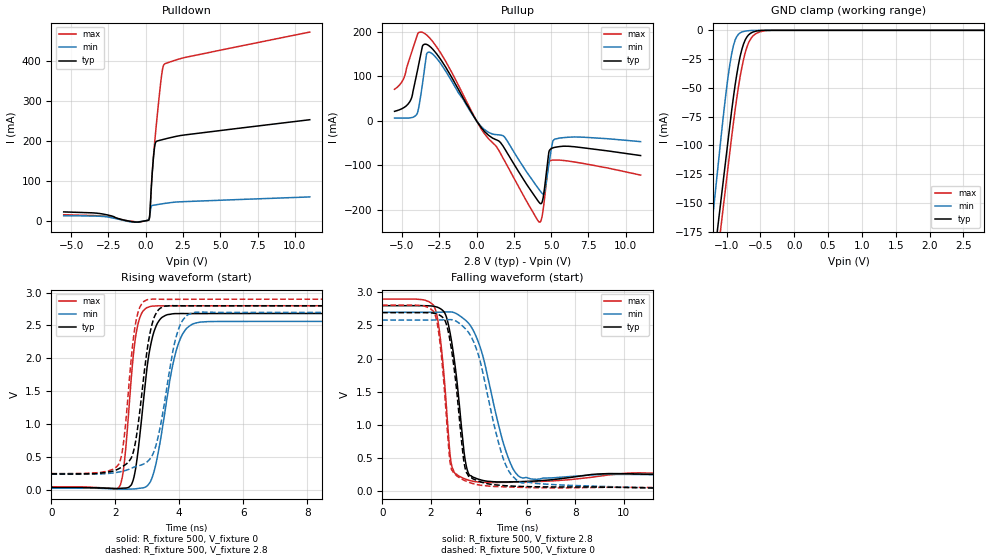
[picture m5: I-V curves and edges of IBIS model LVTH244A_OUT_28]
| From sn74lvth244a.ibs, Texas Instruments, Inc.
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[Model]   LVTH244A_OUT_28
Model_type  3-state
Enable   Active-Low
Vref =   0
Rref =   500
Cref =   50p
Vmeas =   1.5
| variable   typ   min   max
C_comp   5.78pF   4.77pF   7.95pF
| C_pullup   4.85pF   0.29pF   7.49pF
| C_pulldown   5.95pF   2.16pF   9.97pF
| C_tri-state   5.78pF   4.77pF   7.95pF
[Temperature Range]   40   -40   100
| Ambient temperature   25   -40   85
[Voltage range]   2.8   2.7   2.9
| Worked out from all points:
|   slope of the pulldown table from 0 to 0.42 V, typ, clamps not added: 3.84 ohm
|   slope of the pullup table from 0 to 0.42 V, typ, clamps not added: 21.7 ohm
|   GND clamp passes 1 mA (typ) near -0.58 V on its own axis
|   rising waveform, R_fixture 500, V_fixture 0: 20-80 % time 381ps typ, 543ps min, 293ps max; typ from 0.032 V to 2.68 V
|   falling waveform, R_fixture 500, V_fixture 2.8: 20-80 % time 483ps typ, 987ps min, 372ps max; typ from 2.8 V to 0.238 V
|   rising waveform, R_fixture 500, V_fixture 2.8: 20-80 % time 408ps typ, 541ps min, 311ps max; typ from 0.238 V to 2.8 V
|   falling waveform, R_fixture 500, V_fixture 0: 20-80 % time 484ps typ, 1ns min, 378ps max; typ from 2.69 V to 0.032 V
[GND Clamp]
| LVTH244A_OUT_28
|   Voltage   I(typ)   I(min)   I(max)
-5.5V     -2.834A    -3.019A    -2.854A
-1.22V    -215.7mA   -171mA     -239.3mA
-1.18V    -195.7mA   -148.2mA   -219mA
-1.075V   -143.6mA   -88.89mA   -166.6mA
-975mV    -94.01mA   -38.86mA   -117.1mA
-925mV    -69.63mA   -20.27mA   -92.47mA
-875mV    -47.88mA   -8.568mA   -69.46mA
-800mV    -22.55mA   -2.203mA   -40.18mA
-725mV    -8.33mA    -701.6uA   -19.48mA
-650mV    -2.727mA   -178.1uA   -7.97mA
-575mV    -842.6uA   -11.41uA   -3.176mA
2.8V      28.19pA    20.95pA    1.193nA
[Pulldown]
| LVTH244A_OUT_28
|   Voltage   I(typ)   I(min)   I(max)
-5.5V     21.78mA    11.95mA    14.77mA
-3.075V   17.71mA    10.9mA     12.09mA
-725mV    -3.49mA    -3.914mA   -2.787mA
215mV     2.328mA    2.63mA     2.413mA
285mV     22.67mA    17.43mA    18.31mA
365mV     76.4mA     34.4mA     76.07mA
465mV     132.9mA    38.15mA    135.3mA
620mV     189.6mA    39.16mA    203.7mA
1.05V     201.9mA    41.75mA    359.1mA
1.155V    202.9mA    42.35mA    383.6mA
1.26V     203.9mA    42.94mA    391.5mA
11V       252.3mA    59.26mA    471.4mA
[Pullup]
| LVTH244A_OUT_28
|   Voltage   I(typ)   I(min)   I(max)
-5.5V     21.44mA    6.413mA    70.85mA
-4.465V   43.68mA    6.74mA     142.4mA
-3.99V    108.8mA    16.01mA    191mA
-3.62V    168.2mA    84.82mA    198.4mA
-3.245V   169.8mA    153.9mA    189.4mA
1.895V    -62.93mA   -36.94mA   -90.63mA
4.215V    -183.5mA   -154.8mA   -227.1mA
4.55V     -152.6mA   -160.2mA   -176.4mA
4.815V    -78.5mA    -105.1mA   -97.39mA
4.96V     -63.26mA   -73.72mA   -89.02mA
5.57V     -57.52mA   -38.52mA   -87.94mA
11V       -77.73mA   -46.53mA   -121.5mA
[Ramp]
| LVTH244A_OUT_28
| variable   typ   min   max
dV/dt_r   1.60/3.90E-10   1.53/5.56E-10   1.67/2.99E-10
dV/dt_f   1.60/4.99E-10   1.51/1.03E-09   1.67/3.85E-10
R_load = 500
[Rising Waveform]
| LVTH244A_OUT_28
R_fixture =   500
C_fixture =   0
L_fixture =   0
V_fixture =   0
V_fixture_min = 0
V_fixture_max = 0
|   Time   V(typ)   V(min)   V(max)
0s        32.2mV     21.67mV    40.66mV
2.15ns    17.78mV    6.769mV    62.49mV
2.29ns    21.9mV     5.581mV    446.6mV
2.51ns    80.48mV    7.332mV    1.761V
2.665ns   413.2mV    13.11mV    2.416V
3.145ns   2.289V     173.6mV    2.794V
3.43ns    2.61V      804.9mV    2.798V
3.935ns   2.68V      2.164V     2.799V
4.675ns   2.681V     2.552V     2.8V
50ns      2.684V     2.563V     2.801V
[Falling Waveform]
| LVTH244A_OUT_28
R_fixture =   500
C_fixture =   0
L_fixture =   0
V_fixture =   2.8
V_fixture_min = 2.7
V_fixture_max = 2.9
|   Time   V(typ)   V(min)   V(max)
0s        2.8V       2.7V       2.9V
2.125ns   2.791V     2.701V     2.807V
2.35ns    2.766V     2.702V     2.466V
2.59ns    2.689V     2.704V     1.602V
2.895ns   2.205V     2.704V     352.3mV
3.445ns   442.5mV    2.581V     173.7mV
3.825ns   194.9mV    2.386V     137.4mV
5.11ns    131.9mV    609mV      125mV
5.81ns    137.3mV    191.3mV    130mV
50ns      237.6mV    232.9mV    243.3mV
[Rising Waveform]
| LVTH244A_OUT_28
R_fixture =   500
C_fixture =   0
L_fixture =   0
V_fixture =   2.8
V_fixture_min = 2.7
V_fixture_max = 2.9
|   Time   V(typ)   V(min)   V(max)
0s        238mV      233.1mV    243.6mV
2.115ns   318.4mV    267mV      391.1mV
2.27ns    364mV      283.8mV    766.3mV
2.515ns   500.3mV    327.6mV    2.079V
2.64ns    749.6mV    349.4mV    2.547V
3.04ns    2.265V     442mV      2.897V
3.345ns   2.735V     814.1mV    2.9V
3.94ns    2.801V     2.387V     2.898V
4.51ns    2.798V     2.701V     2.899V
50ns      2.8V       2.7V       2.9V
[Falling Waveform]
| LVTH244A_OUT_28
R_fixture =   500
C_fixture =   0
L_fixture =   0
V_fixture =   0
V_fixture_min = 0
V_fixture_max = 0
|   Time   V(typ)   V(min)   V(max)
0s        2.695V     2.582V     2.808V
2.12ns    2.687V     2.583V     2.716V
2.34ns    2.663V     2.584V     2.389V
2.575ns   2.591V     2.586V     1.526V
2.87ns    2.13V      2.588V     320mV
3.43ns    345.6mV    2.456V     149.4mV
4.06ns    134.5mV    1.953V     82.34mV
4.995ns   76.7mV     501.6mV    57.39mV
5.825ns   62.26mV    114.4mV    48.55mV
50ns      32.23mV    21.69mV    40.72mV
